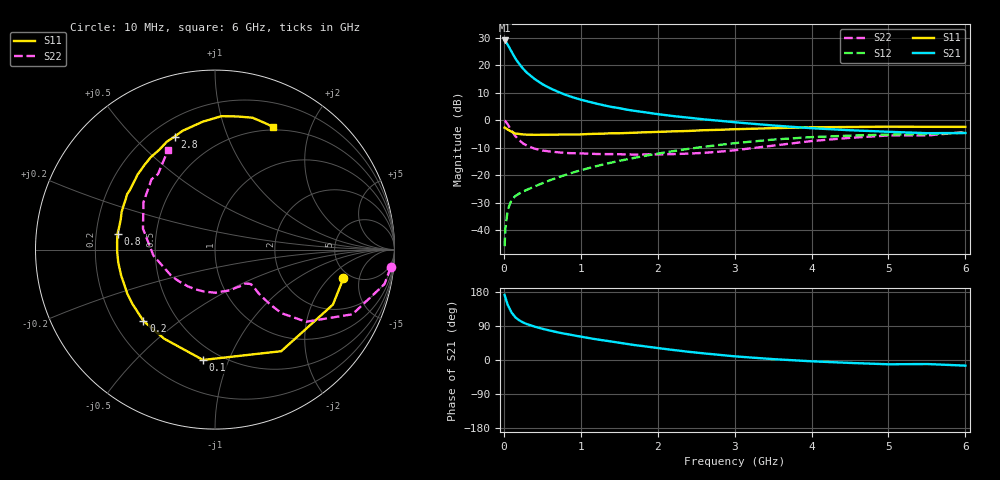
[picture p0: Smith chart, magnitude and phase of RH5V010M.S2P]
! SIEMENS Small Signal Semiconductors
! BFR106
! Si NPN RF Bipolar Junction Transistor in SOT23
! VCE = 5 V  IC = 10 mA
! Common Emitter S-Parameters:  August  1996
# GHz  S  MA  R  50
!  f  S11  S21  S12  S22
! GHz  MAG  ANG  MAG  ANG  MAG  ANG  MAG  ANG
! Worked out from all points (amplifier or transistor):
!   36 points, 10 MHz to 6 GHz, reference 50 ohm
!   highest |S21| = 29.0 dB at 10 MHz (marker M1)
!   |S21| within 3 dB of that: start of sweep to 79.04 MHz
!   unconditionally stable (mu >= 1): 485.1 MHz to 1.986 GHz; 5.309 GHz to end of sweep
!   at 250 MHz: K = 0.71, MSG = 22.4 dB, |S12| = -26.0 dB
!   at 1.4 GHz: K = 1.08, MAG = 8.4 dB, |S12| = -15.4 dB
!   at 6 GHz: K = 1.01, MAG = -0.5 dB, |S12| = -4.6 dB
!   S11 on the Smith chart (normalised r, x): 10 MHz: 4.34, -3.00; 100 MHz: 0.41, -0.81; 200 MHz: 0.32, -0.38; 800 MHz: 0.29, +0.07; 2.8 GHz: 0.29, +0.66; 6 GHz: 0.46, +1.48
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0.01  0.7331 -12.6  28.3 171.6  0.0051 86.1  0.9838 -5.8
0.02  0.725 -25.0  27.58 164.9  0.0107 79.0  0.9638 -11.5
0.05  0.6757 -56.9  23.76 145.7  0.0232 65.0  0.8464 -25.2
0.1  0.6184 -96.2  17.71 125.4  0.0355 51.9  0.6473 -38.4
0.15  0.5715 -119.7  13.29 112.6  0.0417 47.5  0.5128 -43.7
0.2  0.5629 -135.1  10.59 104.9  0.0463 47.2  0.4336 -44.8
0.25  0.5508 -146.5  8.676 98.9  0.0503 47.6  0.3773 -45.1
0.3  0.5469 -153.3  7.338 94.8  0.0542 49.3  0.3454 -45.1
0.4  0.5424 -164.6  5.625 88.1  0.0624 52.7  0.3036 -44.1
0.5  0.5439 -172.6  4.537 82.5  0.0712 55.5  0.2813 -43.8
0.6  0.5454 -179.4  3.827 77.6  0.0808 58.0  0.2693 -44.9
0.8  0.55 170.7  2.908 69.1  0.101 60.9  0.2535 -48.4
0.9  0.5485 166.3  2.603 65.3  0.112 61.7  0.2507 -50.4
1.1  0.5608 158.1  2.176 58.1  0.134 62.8  0.2462 -56.8
1.3  0.5702 151.1  1.87 51.7  0.1578 62.6  0.2416 -63.4
1.6  0.5855 141.4  1.554 42.5  0.1941 61.5  0.2386 -75.5
2.2  0.627 124.8  1.191 26.5  0.2738 56.1  0.2418 -104.0
2.8  0.6685 109.7  0.978 13.6  0.3548 47.8  0.2673 -138.6
3.5  0.7162 95.4  0.802 2.3  0.4442 36.4  0.3446 -174.4
4.5  0.7526 80.2  0.657 -7.7  0.5244 18.9  0.4778 146.5
5.5  0.7581 68.4  0.581 -10.6  0.5593 7.1  0.527 127.1
6  0.7564 64.5  0.585 -14.9  0.5906 -0.7  0.6118 115.4
